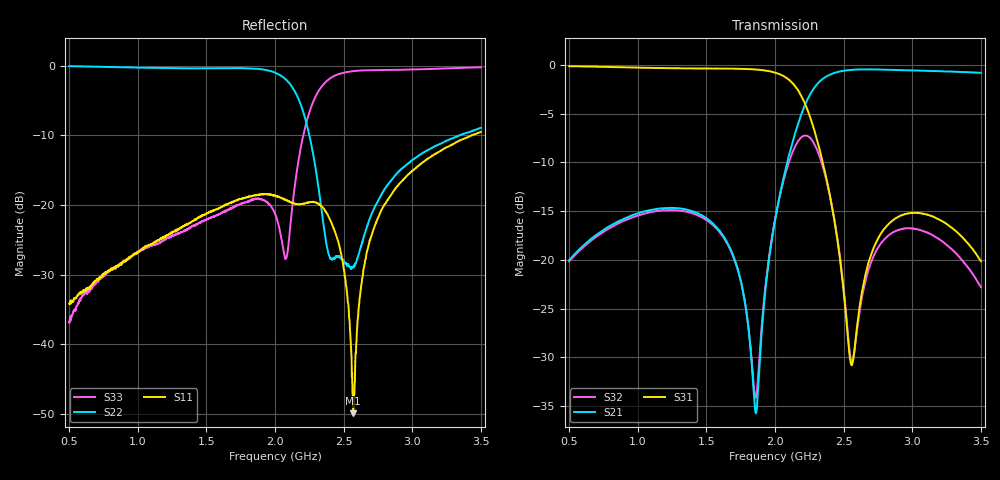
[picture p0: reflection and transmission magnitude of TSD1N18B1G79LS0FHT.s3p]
# MHZ S RI R 50
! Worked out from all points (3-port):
!   1501 points, 500 MHz to 3.5 GHz, reference 50 ohm
!   strongest paths, dB at 500 MHz, 1.25 GHz, 2 GHz, 2.75 GHz, 3.5 GHz:
!     S31: -0.1, -0.3, -0.8, -17.8, -20.1
!     S21: -20.0, -14.7, -16.0, -0.5, -0.8
!     S32: -20.2, -14.9, -15.9, -18.8, -22.8
!   lowest |S11| = -49.9 dB at 2.57 GHz (marker M1), VSWR 1.01, Z = 50 + j0.319 ohm
!   |S11| at or under -10 dB: start of sweep to 3.433 GHz
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500  0.00862 -0.0176  0.029 0.0956  0.9409 -0.3012
     0.0286 0.0954  0.8759 -0.4695  0.0492 0.0846
     0.9399 -0.3008  0.0494 0.0849  -0.0137 -0.00432
1518  -0.0201 -0.0862  0.1314 0.0912  0.4656 -0.8388
      0.1315 0.0909  -0.0698 -0.957  0.1531 -0.0336
      0.465 -0.839  0.153 -0.0338  -0.0688 0.0412
1860  -0.0616 -0.0997  -0.00152 0.0163  0.0391 -0.9478
      -0.00146 0.0162  -0.6325 -0.7135  0.0171 0.00912
      0.0389 -0.9481  0.0174 0.00922  -0.0737 0.0821
2000  -0.0784 -0.0866  -0.1561 0.0319  -0.2427 -0.8818
      -0.1557 0.0316  -0.8234 -0.3474  0.0329 0.1572
      -0.242 -0.8823  0.0328 0.1575  -0.018 0.0849
2084  -0.0792 -0.074  -0.2888 0.1031  -0.4273 -0.7447
      -0.2883 0.1033  -0.7889 -0.0226  0.1634 0.2395
      -0.4272 -0.745  0.1633 0.24  0.0419 0.00484
2254  -0.0806 -0.0676  -0.4292 0.5578  -0.5043 -0.2078
      -0.429 0.557  -0.1863 0.2411  0.4116 -0.1001
      -0.5043 -0.2078  0.4123 -0.1  -0.3386 -0.3338
2418  -0.0706 -0.0136  -0.0734 0.9009  -0.1824 0.00301
      -0.073 0.9007  -0.041 -0.00261  0.0574 -0.1746
      -0.1828 0.00288  0.0575 -0.1748  -0.7828 0.2817
2570  0.000139 0.00319  0.2543 0.9113  -0.00345 -0.0307
      0.2541 0.9112  -0.00514 -0.0357  0.0303 -0.00721
      -0.00365 -0.0306  0.0304 -0.00707  -0.4947 0.7705
2774  0.0803 -0.044  0.5254 0.7897  0.0727 -0.1161
      0.5249 0.7894  0.0727 -0.0938  0.1182 0.029
      0.073 -0.1162  0.1186 0.0292  -0.000276 0.9324
3500  0.1095 -0.3171  0.8532 0.3237  -0.0221 -0.0963
      0.8531 0.3242  0.1163 -0.3389  0.0606 -0.0402
      -0.0222 -0.0959  0.0603 -0.0401  0.8985 0.3809
